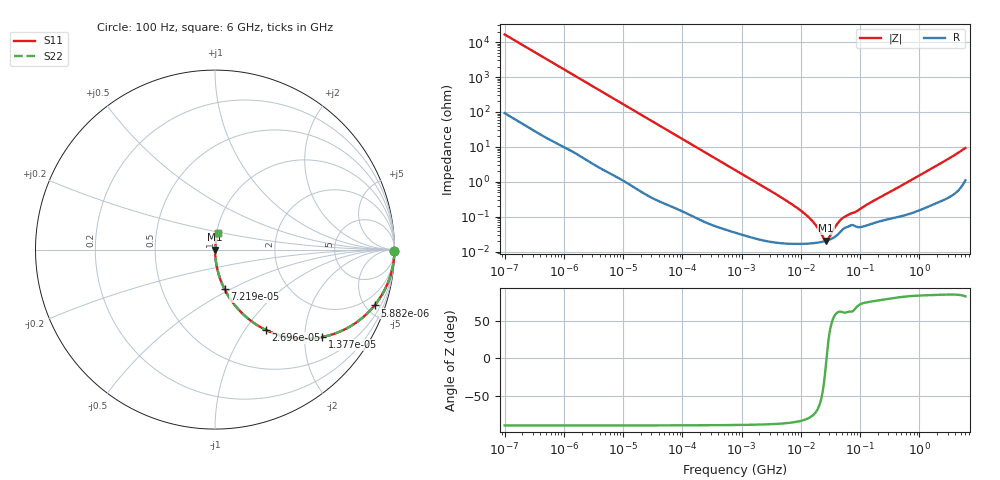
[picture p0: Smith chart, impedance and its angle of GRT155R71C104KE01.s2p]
!Murata Part Number: GRT155R71C104KE01
!These Parameters are Measured in Series Mode Connection
!Data Generated on Jun 19, 2026
!  o--ll--o
!Port1  Port2
!  o------o
!Operation Temp=25[degC], DC Bias Voltage=0[V]
!Freq. Start=100[Hz] Stop=6[GHz] 401[Steps]
# Hz S RI R 50
!Freq.(Hz) S11(Real) S11(Imag) S21(Real) S21(Imag) S12(Real) S12(Imag) S22(Real) S22(Imag)
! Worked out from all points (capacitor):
!   401 points, 100 Hz to 6 GHz, reference 50 ohm
!   read as one part in series: C = 96.3 nF near 109 Hz
!   lowest |Z| = 20.7 mohm at 26.62 MHz (marker M1)
!   series resonance near 27.16 MHz, so ESL is about 360 pH
!   S11 on the Smith chart (normalised r, x): 100 Hz: open; 5.882 kHz: 1.04, -5.70; 13.77 kHz: 1.02, -2.44; 26.96 kHz: 1.01, -1.25; 72.19 kHz: 1.00, -0.47; 6 GHz: 1.02, +0.19
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100  0.9999 -0.00606  7.09e-05 0.00606  7.09e-05 0.00606  0.9999 -0.00606
627  0.9984 -0.0377  0.00164 0.0377  0.00164 0.0377  0.9984 -0.0377
2008  0.985 -0.1185  0.015 0.1185  0.015 0.1185  0.985 -0.1185
5882  0.8887 -0.3114  0.1113 0.3114  0.1113 0.3114  0.8887 -0.3114
8801  0.7827 -0.4092  0.2173 0.4092  0.2173 0.4092  0.7827 -0.4092
13772  0.5978 -0.4871  0.4022 0.4871  0.4022 0.4871  0.5978 -0.4871
26957  0.2822 -0.447  0.7178 0.447  0.7178 0.447  0.2822 -0.447
40335  0.1506 -0.3543  0.8494 0.3543  0.8494 0.3543  0.1506 -0.3543
72189  0.0536 -0.2213  0.9464 0.2213  0.9464 0.2213  0.0536 -0.2213
193316  0.00849 -0.0871  0.9915 0.0871  0.9915 0.0871  0.00849 -0.0871
774597  0.00084 -0.0221  0.9992 0.0221  0.9992 0.0221  0.00084 -0.0221
6644369  0.000175 -0.00245  0.9998 0.00245  0.9998 0.00245  0.000175 -0.00245
1.087309e7  0.000171 -0.00134  0.9998 0.00134  0.9998 0.00134  0.000171 -0.00134
1.555665e7  0.000176 -0.000749  0.9998 0.000749  0.9998 0.000749  0.000176 -0.000749
1.86079e7  0.000181 -0.000495  0.9998 0.000495  0.9998 0.000495  0.000181 -0.000495
2.434276e7  0.000198 -0.000141  0.9998 0.000141  0.9998 0.000141  0.000198 -0.000141
2.662322e7  0.000206 -2.54e-05  0.9998 2.54e-05  0.9998 2.54e-05  0.000206 -2.54e-05
2.911731e7  0.000216 8.98e-05  0.9998 -8.98e-05  0.9998 -8.98e-05  0.000216 8.98e-05
3.983537e7  0.000288 0.000508  0.9997 -0.000508  0.9997 -0.000508  0.000288 0.000508
5.211241e7  0.000452 0.000837  0.9995 -0.000837  0.9995 -0.000837  0.000452 0.000837
3.124326e8  0.000895 0.00497  0.9991 -0.00497  0.9991 -0.00497  0.000895 0.00497
6e9  0.0193 0.0901  0.9807 -0.0901  0.9807 -0.0901  0.0193 0.0901
